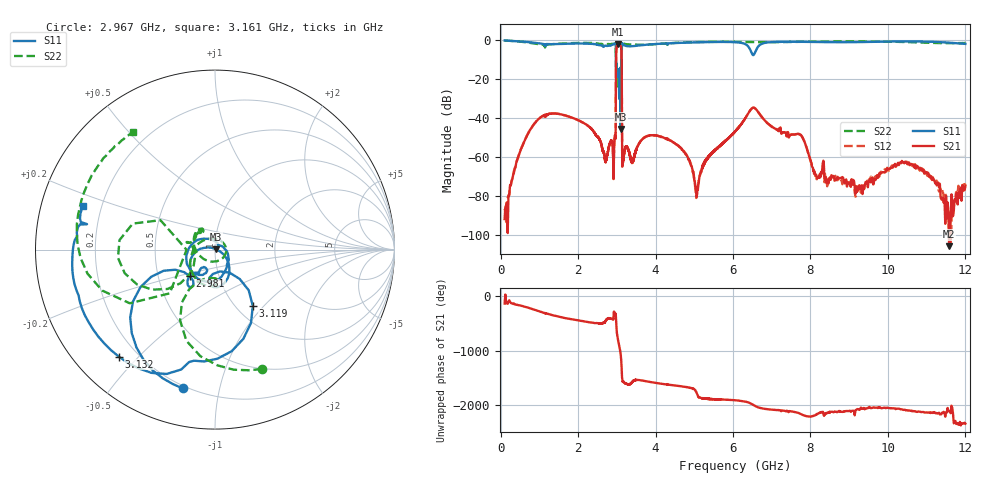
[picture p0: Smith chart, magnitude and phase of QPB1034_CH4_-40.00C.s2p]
! TDS: k:\Engsetup\Winsaw\QPB1034_ALL
! Channel 1
! Ports=1 2
! seg 1=100.000000 1100.000000 51
! seg 2=1101.000000 1301.000000 201
! seg 3=1302.000000 2302.000000 101
! seg 4=2303.000000 3503.000000 1201
! seg 5=3504.000000 5204.000000 171
! seg 6=5205.000000 6405.000000 1201
! seg 7=6406.000000 8506.000000 211
! seg 8=8507.000000 12007.000000 176
! Points=3313
! FailCode=0
! Topology=ALL_SE(12)
!VNA Cal loaded =QPB1034_ALL_-40C
!PS1(V)= 5.000
!PS(mA)= 0.429
!PS2(V)= 1.170
!PS(mA)= -0.001
!PS3(V)= 0.630
!PS(mA)= 0.000
!PS4(V)= 0.630
!PS(mA)= -0.001
!Temp (C)= -40.00
# MHz S DB R 50
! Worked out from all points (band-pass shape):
!   3313 points, 100 MHz to 12.01 GHz, reference 50 ohm
!   highest |S21| = -2.26 dB at 3.033 GHz (marker M1); lowest = -106.0 dB at 11.59 GHz (marker M2)
!   |S21| within 3 dB of the highest: 2.987 GHz to 3.118 GHz (131.3 MHz wide, 4.3 % of centre)
!   lowest |S11| = -45.7 dB at 3.099 GHz (marker M3), VSWR 1.01, Z = 50.5 + j0.165 ohm
!   |S11| at or under -10 dB: 2.978 GHz to 3.118 GHz (140.4 MHz wide, 4.61 % of centre)
!   |S22| runs from -24.6 to -0.3 dB; largest |S21 - S12| = 0.0046
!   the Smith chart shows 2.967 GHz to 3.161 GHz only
!   S11 on the Smith chart (normalised r, x): 2.967 GHz: 0.19, -0.78; 2.981 GHz: 0.73, -0.23; 3.119 GHz: 1.19, -0.87; 3.132 GHz: 0.13, -0.44; 3.161 GHz: 0.13, +0.16
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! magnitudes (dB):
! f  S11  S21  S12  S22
! 100 MHz  -0.3  -92.0  -86.7  -0.3
! 240 MHz  -0.4  -74.6  -75.2  -0.5
! 500 MHz  -0.8  -57.4  -57.2  -0.9
! 1.1 GHz  -2.0  -38.9  -39.0  -2.4
! 2.434 GHz  -2.2  -48.0  -48.1  -1.6
! 2.913 GHz  -2.2  -68.4  -68.8  -2.0
! 2.967 GHz  -2.0  -49.9  -49.8  -2.9
! 2.981 GHz  -13.8  -8.3  -8.3  -15.7
! 3.033 GHz  -15.1  -2.3  -2.3  -17.9
! 3.099 GHz  -45.7  -3.0  -3.0  -17.9
! 3.119 GHz  -8.5  -5.9  -5.9  -7.6
! 3.132 GHz  -1.9  -37.8  -37.8  -2.3
! 3.161 GHz  -2.2  -61.9  -62.0  -2.0
! 3.914 GHz  -2.2  -49.0  -48.9  -2.3
! 5.064 GHz  -1.2  -80.6  -80.3  -1.1
! 5.406 GHz  -1.1  -59.1  -58.9  -1.0
! 6.556 GHz  -7.1  -34.9  -34.9  -1.1
! 7.726 GHz  -0.9  -48.6  -48.5  -1.0
! 8.286 GHz  -1.1  -69.0  -69.1  -0.8
! 10.51 GHz  -0.7  -63.8  -62.7  -1.1
! 11.59 GHz  -1.4  -106.0  -101.6  -1.7
! 12.01 GHz  -2.0  -75.1  -73.8  -1.5
